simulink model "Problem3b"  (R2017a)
settings: Solver=ode1  StartTime=0.0  StopTime=100  FixedStep=0.01  RelTol=1e-3
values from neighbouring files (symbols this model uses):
  kp = 0.851    [Problem3.m]
  Kp = 5    [Problem3.m]
  noise_var = 0.01    [Problem3.m]
  SP = 0    [Problem3.m]
  T = 10    [Problem3.m]
  tau = 2    [Problem3.m]
  tauf = 1    [Problem3.m]
  Td = 1.375    [Problem3.m]
  Ti = 5.5    [Problem3.m]

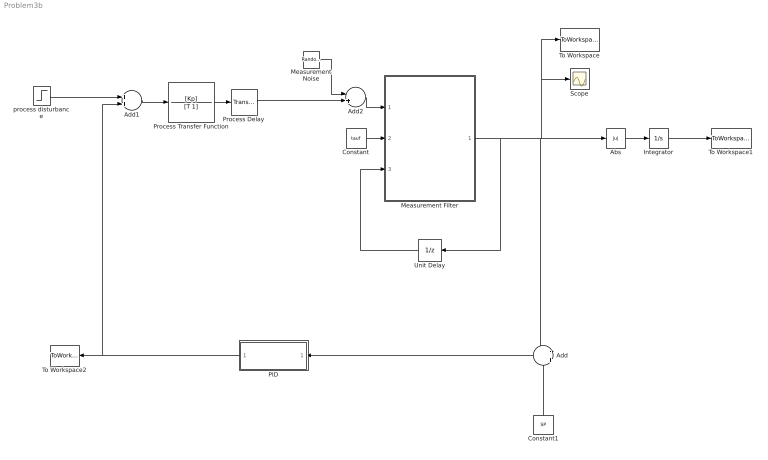
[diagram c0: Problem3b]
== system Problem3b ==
  Abs : Abs
  Add : Sum  Inputs=-+
  Add1 : Sum
  Add2 : Sum  Inputs=-+
  Constant : Constant  Value=tauf
  Constant1 : Constant  Value=SP
  Integrator : Integrator
  Measurement Noise : RandomNumber  Variance=noise_var  SampleTime=0.1
  Measurement Filter : MATLAB Function  TreatAsAtomicUnit=on
  PID : Subsystem
  Process Delay : TransportDelay  DelayTime=tau
  Process Transfer Function : TransferFcn  Numerator=[Kp]  Denominator=[T 1]
  Scope : Scope
  To Workspace : ToWorkspace  VariableName=y_mf  SampleTime=-1
  To Workspace1 : ToWorkspace  VariableName=IAE  SampleTime=-1
  To Workspace2 : ToWorkspace  VariableName=u  SampleTime=-1
  Unit Delay : UnitDelay  SampleTime=0.01
  process disturbance : Step  Time=10  SampleTime=0
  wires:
  Process Transfer Function/1 -> Process Delay/1
  Process Delay/1 -> Add2/2
  Constant/1 -> Measurement Filter/2(tau)
  Measurement Filter/1(ymeas) -> To Workspace/1, Scope/1, Abs/1, Add/1, Unit Delay/1
  Unit Delay/1 -> Measurement Filter/3(ut2)
  Constant1/1 -> Add/2
  PID/1(Out1) -> Add1/2, To Workspace2/1
  process disturbance/1 -> Add1/1
  Add1/1 -> Process Transfer Function/1
  Add/1 -> PID/1(In1)
  Abs/1 -> Integrator/1
  Integrator/1 -> To Workspace1/1
  Measurement Noise/1 -> Add2/1
  Add2/1 -> Measurement Filter/1(ut1)

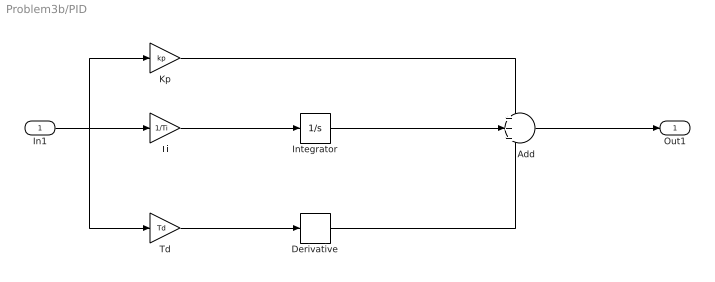
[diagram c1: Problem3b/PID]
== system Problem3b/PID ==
  In1 : Inport
  Add : Sum  Inputs=+++
  Derivative : Derivative
  Integrator : Integrator
  Kp : Gain  Gain=kp
  Td : Gain  Gain=Td
  Ti : Gain  Gain=1/Ti
  Out1 : Outport
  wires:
  In1/1 -> Kp/1, Td/1, Ti/1
  Kp/1 -> Add/1
  Ti/1 -> Integrator/1
  Td/1 -> Derivative/1
  Integrator/1 -> Add/2
  Derivative/1 -> Add/3
  Add/1 -> Out1/1

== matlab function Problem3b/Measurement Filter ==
function ymeas = fcn(ut1,tau, ut2)
alpha = 0.01/(tau+0.01);
ymeas = alpha*ut1+(1-alpha)*ut2;
